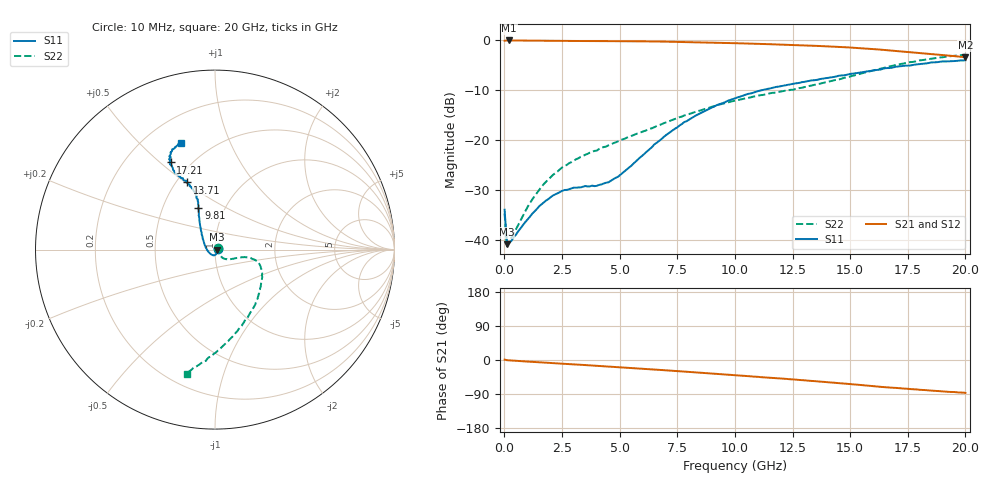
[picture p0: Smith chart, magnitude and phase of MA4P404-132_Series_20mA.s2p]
! AWR Design Environment (9226) Thu Aug 19 02:30:18 2021
! Document = '20mA'
! nPorts: 2, nXvals: 201
# GHz S DB R 50
!Freq DBS11 AngS11 DBS21 AngS21 DBS12 AngS12 DBS22 AngS22
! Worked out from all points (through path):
!   201 points, 10 MHz to 20 GHz, reference 50 ohm
!   highest |S21| = -0.13 dB at 210 MHz (marker M1); lowest = -3.5 dB at 20 GHz (marker M2)
!   group delay of S21, straight-line fit = 12.2 ps
!   lowest |S11| = -40.9 dB at 110 MHz (marker M3), VSWR 1.02, Z = 50.9 - j0.102 ohm
!   |S11| at or under -10 dB: start of sweep to 11.24 GHz
!   |S22| runs from -41.3 to -3.0 dB; largest |S21 - S12| = 0.034
!   S11 on the Smith chart (normalised r, x): 10 MHz: 1.04, +0.01; 9.81 GHz: 0.75, +0.37; 13.71 GHz: 0.57, +0.51; 17.21 GHz: 0.39, +0.54; 20 GHz: 0.35, +0.67
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0.01  -34.01 15.5  -0.20 1.0  -0.18 0.7  -34.75 35.7
0.11  -40.94 -6.4  -0.13 -0.5  -0.12 -0.5  -41.30 -7.1
0.21  -40.70 -11.8  -0.13 -0.9  -0.12 -0.9  -40.30 -10.3
1.11  -35.39 -53.8  -0.17 -4.6  -0.15 -4.4  -32.66 -41.0
1.71  -32.57 -70.6  -0.20 -6.8  -0.18 -6.6  -28.88 -46.1
2.51  -30.22 -91.5  -0.23 -9.7  -0.21 -9.4  -25.54 -48.8
3.41  -29.40 -115.9  -0.25 -13.1  -0.23 -12.5  -23.24 -45.5
4.01  -29.23 -135.7  -0.26 -15.3  -0.25 -14.8  -22.17 -41.9
4.91  -27.46 -175.2  -0.28 -18.7  -0.27 -18.1  -20.36 -34.2
6.71  -20.26 135.7  -0.35 -26.0  -0.33 -25.1  -17.09 -18.8
7.81  -16.45 122.8  -0.43 -30.6  -0.43 -29.5  -15.13 -14.0
8.81  -13.96 116.1  -0.54 -34.8  -0.52 -33.6  -13.67 -13.4
9.81  -12.03 111.8  -0.65 -39.1  -0.64 -37.7  -12.41 -15.2
10.01  -11.71 110.5  -0.67 -40.2  -0.66 -38.6  -12.20 -15.4
11.71  -9.52 109.5  -0.91 -47.5  -0.85 -45.8  -10.59 -27.3
13.41  -8.10 112.2  -1.19 -55.4  -1.09 -53.8  -9.05 -46.6
13.71  -7.84 112.7  -1.25 -57.1  -1.15 -55.2  -8.77 -50.5
14.81  -7.05 115.4  -1.49 -62.5  -1.38 -60.8  -7.54 -64.3
16.71  -5.65 117.5  -2.11 -72.7  -2.00 -71.0  -5.34 -85.5
17.21  -5.27 117.0  -2.31 -74.9  -2.21 -73.6  -4.83 -89.6
18.71  -4.49 114.5  -2.93 -81.3  -2.91 -80.8  -3.63 -98.9
20  -4.10 107.6  -3.47 -86.8  -3.58 -85.9  -2.98 -102.9
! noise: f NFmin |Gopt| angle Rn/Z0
0.01  0  1  0  2e-20
2.21  0  1  0  2e-20
4.41  0  1  0  2e-20
6.61  0  1  0  2e-20
8.81  0  1  0  2e-20
11.11  0  1  0  2e-20
13.31  0  1  0  2e-20
15.51  0  1  0  2e-20
17.71  0  1  0  2e-20
20  0  1  0  2e-20
